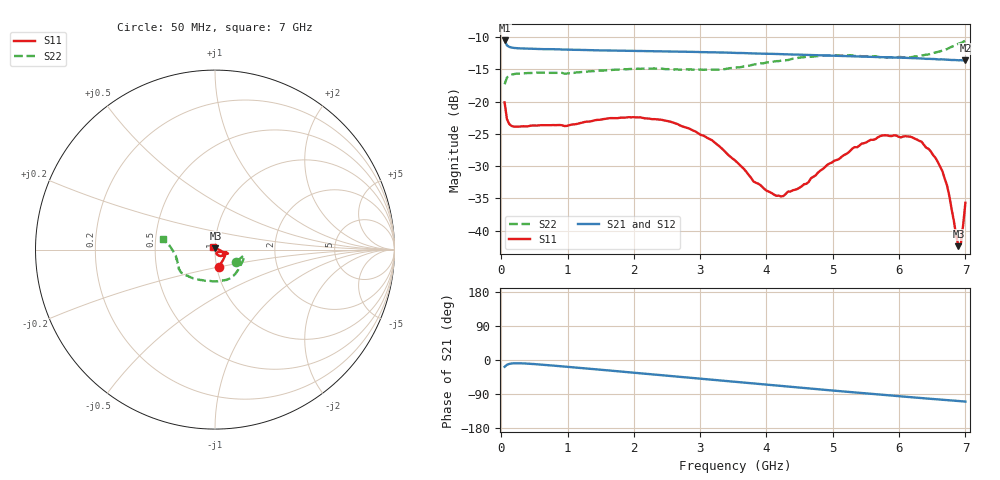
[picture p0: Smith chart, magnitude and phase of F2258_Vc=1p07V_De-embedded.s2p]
! Integrated Device Technology
! Corporate Headquarters
! 6024 Silver Creek Valley Road
! San Jose, CA 95138  USA
! Phone:  1-408-284-8200
! Toll Free:  1-800-223-1366
! Webpage:  http://www.idt.com/
! Timing and RF Division
! 515 Groton Road, Suite 102
! Westford, MA 01886-6024
! Device:  F2258
! Description: Voltage Variable RF Attenuator
! Frequency:  50.0 -  6000.00 MHz
! Package:  3x3 mm Thin QFN Plastic Package: 16 pin
! Ports:  2 RF, 2 DC
!  Pin  1  = NC
!  Pin  2  = NC
!  Pin  3  = RF2  = Port 2
!  Pin  4  = GND
!  Pin  5  = Vdd
!  Pin  6  = NC
!  Pin  7  = VCTRL
!  Pin  8  = NC
!  Pin  9  = GND
!  Pin 10  = RF1  = Port 1
!  Pin 11  = NC
!  Pin 12  = NC
!  Pin 13  = NC
!  Pin 14  = NC
!  Pin 15  = NC
!  Pin 16  = NC
! Vcntrl:  1.070 Volts
! Vdd:  +3.300 Volts
! Current:  1.159 mA
! Data:  The device was measured on a the F2258 evaluation board which has
!  individual transmission lines to the RF pins.  Data was collected
!  using a calibrated network analyzer.  The evaluation board was
!  de-embedded using a TRL calibration technique.
!  The reference plane is the edge of the package pin.
! Misc:  SN 10
!  Action Tracker AT0285
! Date Measured:  2014-12-10
! Date:  2016-01-13  MJV
! Note:
!  Integrated Device Technology supplies this data as a sample of measured
!  data at the package pin for this product.  Your particular data for this
!  product may vary.
!  Data was taken at 25 degrees C.
!  Integrated Device Technology reserves the right to change this data at anytime.
!Freq_(GHz)  S11M_(dB)  S11P_(deg)  S21M_(dB)  S21P_(deg)  S12M_(dB)  S12P_(deg)  S22M_(dB)  S22P_(deg)
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# GHz S dB R 50
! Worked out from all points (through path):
!   201 points, 50 MHz to 7 GHz, reference 50 ohm
!   highest |S21| = -10.52 dB at 50 MHz (marker M1); lowest = -13.6 dB at 7 GHz (marker M2)
!   group delay of S21, straight-line fit = 42.4 ps
!   lowest |S11| = -42.4 dB at 6.896 GHz (marker M3), VSWR 1.02, Z = 50.2 + j0.722 ohm
!   |S11| at or under -10 dB: start of sweep to end of sweep
!   |S22| runs from -17.3 to -10.5 dB; largest |S21 - S12| = 0.0011
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0.05  -20.12 -78.1  -10.52 -18.0  -10.49 -17.9  -17.32 -29.6
0.08475  -22.69 -52.5  -11.27 -12.7  -11.25 -12.7  -16.28 -16.4
0.189  -23.87 -24.8  -11.67 -8.7  -11.66 -8.7  -15.74 -11.7
1.2315  -23.25 -18.0  -11.99 -21.6  -11.96 -21.6  -15.40 -39.2
1.9265  -22.41 -16.8  -12.11 -32.3  -12.12 -32.3  -14.95 -57.1
2.37825  -22.77 -15.5  -12.19 -39.4  -12.20 -39.3  -14.88 -69.1
3.07325  -25.40 -15.5  -12.33 -50.4  -12.32 -50.4  -15.06 -92.2
3.525  -29.10 -20.9  -12.45 -57.7  -12.44 -57.7  -14.75 -110.2
3.803  -32.36 -33.5  -12.53 -62.1  -12.53 -62.1  -14.26 -120.8
4.1505  -34.60 -54.0  -12.62 -67.6  -12.62 -67.6  -13.72 -131.3
4.46325  -33.55 -71.4  -12.70 -72.5  -12.73 -72.5  -13.25 -139.4
4.7065  -31.66 -69.2  -12.79 -76.2  -12.79 -76.2  -13.02 -143.7
5.332  -27.05 -51.6  -12.97 -85.6  -12.97 -85.5  -12.93 -152.9
5.85325  -25.32 -36.3  -13.13 -93.3  -13.14 -93.3  -13.14 -162.8
6.166  -25.43 -28.8  -13.24 -97.9  -13.26 -97.9  -13.13 -170.1
6.33975  -26.22 -22.8  -13.32 -100.5  -13.33 -100.5  -12.86 -175.0
6.54825  -28.72 -14.4  -13.41 -103.5  -13.40 -103.5  -12.39 179.4
6.6525  -30.76 -7.4  -13.45 -105.0  -13.46 -104.9  -12.09 176.6
6.722  -32.95 -0.2  -13.51 -105.9  -13.51 -105.9  -11.86 174.7
6.89575  -42.41 71.7  -13.59 -108.3  -13.58 -108.3  -11.03 171.0
6.9305  -42.12 101.2  -13.57 -108.8  -13.58 -108.8  -10.91 170.6
7  -35.69 133.5  -13.61 -109.7  -13.63 -109.7  -10.54 168.9
